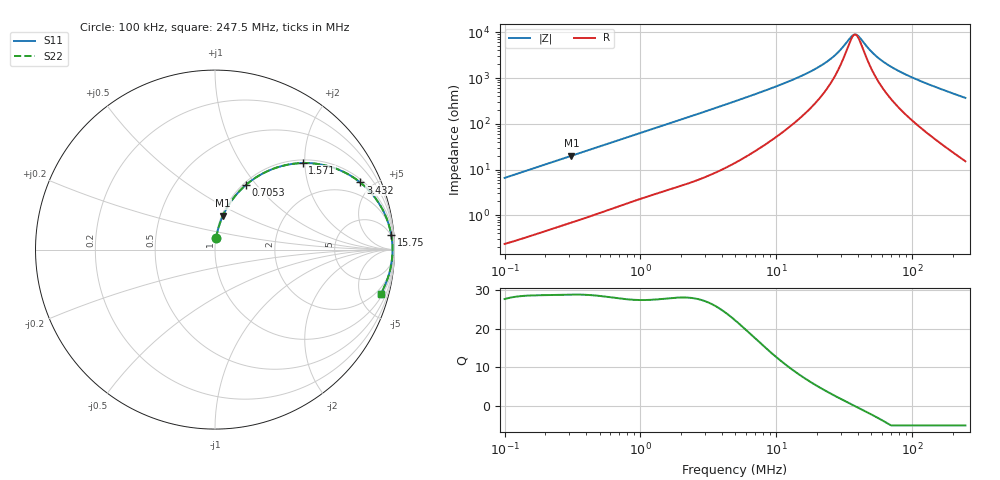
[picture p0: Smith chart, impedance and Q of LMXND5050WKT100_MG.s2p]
! LMXND5050WKT100_MG  S-PARAMETER MODEL  ( General Type )
! Model Generated by TAIYO YUDEN Corporation (http://www.ty-top.com)
! Version 1.0
! TAIYO YUDEN Control No. 191023NI43SB-FBB
! Copyright(c) 2019 TAIYO YUDEN CO.,LTD. All Rights Reserved.
! Product Description (link to TY-COMPAS)
! https://ds.yuden.co.jp/TYCOMPAS/or/detail?pn=LMXND5050WKT100MMG&u=M
! Products Name : Inductors
! Characteristics :
!  Inductance : 10 uH , SRF(min) : 24 MHz , DC Resistance(max) : 0.144 Ohm
!  Rated Current : Saturation :1300 mA , Temp Rise : 1450 mA
!  Case Size : 4.9 x 4.9 / 0.193 x 0.193 [mm/inch] , Thickness : 2 / 0.079 [mm/inch]
!  (Conditions: Temperature = 25 degC , DC Bias Current/Voltage = 0A / 0V)
! External Node Assignments :
!  1  o---GGG---o  2
! GND o---------o GND
! Frequency Range : 0.1MHz  -  247.502633MHz  [ 402 STEP ]
# MHz S RI R 50
! Freq[MHz].  S11 Real  S11 Imag  S21 Real  S21 Imag  S12 Real  S12 Imag  S22 Real  S22 Imag
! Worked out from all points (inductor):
!   401 points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, 100 kHz to 247.5 MHz, reference 50 ohm
!   read as one part in series: L = 10.4 uH near 104 kHz
!   highest Q = 28.9 at 310.5 kHz (marker M1), where L = 10.2 uH
!   self-resonance near 37.94 MHz
!   S11 on the Smith chart (normalised r, x): 100 kHz: 1.00, +0.13; 705.3 kHz: 1.03, +0.89; 1.571 MHz: 1.07, +1.95; 3.432 MHz: 1.16, +4.25; 15.75 MHz: 4, +23; 247.5 MHz: 1.30, -7.35
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0.1  0.0066 0.0649  0.9934 -0.0649  0.9934 -0.0649  0.0066 0.0649
0.310505  0.0443 0.1893  0.9557 -0.1893  0.9557 -0.1893  0.0443 0.1893
0.37019  0.0601 0.2209  0.9399 -0.2209  0.9399 -0.2209  0.0601 0.2209
0.705334  0.1744 0.3619  0.8256 -0.3619  0.8256 -0.3619  0.1744 0.3619
1.370406  0.4242 0.4765  0.5758 -0.4765  0.5758 -0.4765  0.4242 0.4765
1.57122  0.4884 0.4822  0.5116 -0.4822  0.5116 -0.4822  0.4884 0.4822
2.233305  0.6512 0.4591  0.3488 -0.4591  0.3488 -0.4591  0.6512 0.4591
3.432376  0.8095 0.3741  0.1905 -0.3741  0.1905 -0.3741  0.8095 0.3741
4.974964  0.8954 0.2844  0.1046 -0.2844  0.1046 -0.2844  0.8954 0.2844
9.47895  0.9635 0.1539  0.0365 -0.1539  0.0365 -0.1539  0.9635 0.1539
15.75226  0.9816 0.0835  0.0184 -0.0835  0.0184 -0.0835  0.9816 0.0835
18.41681  0.9843 0.0662  0.0157 -0.0662  0.0157 -0.0662  0.9843 0.0662
26.17735  0.9878 0.0322  0.0122 -0.0322  0.0122 -0.0322  0.9878 0.0322
30.01327  0.9885 0.0202  0.0115 -0.0202  0.0115 -0.0202  0.9885 0.0202
35.78235  0.9889 0.0053  0.0111 -0.0053  0.0111 -0.0053  0.9889 0.0053
37.94204  0.989 0.000384  0.011 -0.000384  0.011 -0.000384  0.989 0.000384
41.02574  0.9889 -0.00617  0.0111 0.00617  0.0111 0.00617  0.9889 -0.00617
47.9654  0.9886 -0.0194  0.0114 0.0194  0.0114 0.0194  0.9886 -0.0194
53.93017  0.9881 -0.0297  0.0119 0.0297  0.0119 0.0297  0.9881 -0.0297
68.1772  0.9863 -0.0514  0.0137 0.0514  0.0137 0.0514  0.9863 -0.0514
115.5329  0.9762 -0.1118  0.0238 0.1118  0.0238 0.1118  0.9762 -0.1118
247.5026  0.9223 -0.2479  0.0777 0.2479  0.0777 0.2479  0.9223 -0.2479
